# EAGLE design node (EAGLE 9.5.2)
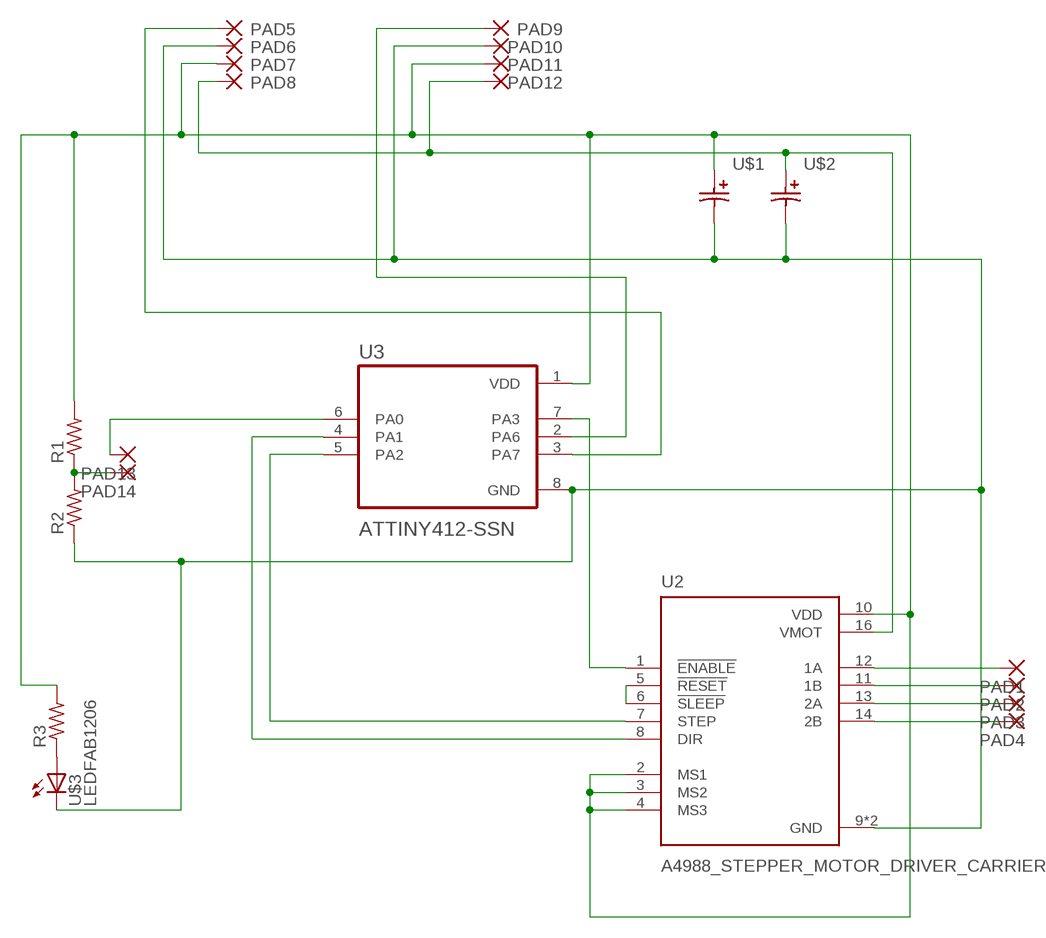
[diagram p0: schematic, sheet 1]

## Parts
PAD1  SMD2  [SMD1,27-2,54]
PAD2  SMD2  [SMD1,27-2,54]
PAD3  SMD2  [SMD1,27-2,54]
PAD4  SMD2  [SMD1,27-2,54]
PAD5  SMD2  [SMD1,27-2,54]
PAD6  SMD2  [SMD1,27-2,54]
PAD7  SMD2  [SMD1,27-2,54]
PAD8  SMD2  [SMD1,27-2,54]
PAD9  SMD2  [SMD1,27-2,54]
PAD10  SMD2  [SMD1,27-2,54]
PAD11  SMD2  [SMD1,27-2,54]
PAD12  SMD2  [SMD1,27-2,54]
PAD13  SMD2  [SMD1,27-2,54]
PAD14  SMD2  [SMD1,27-2,54]
R1  R1206FAB  [R1206FAB]
R2  R1206FAB  [R1206FAB]
R3  R1206FAB  [R1206FAB]
U2  A4988_STEPPER_MOTOR_DRIVER_CARRIER  [MODULE_A4988_STEPPER_MOTOR_DRIVER_CARRIER]
U3  ATTINY412-SSN  [SOIC127P600X175-8N]
U$1  CAP_POLARIZED  [SMD-ELEC-CAP]
U$2  CAP_POLARIZED  [SMD-ELEC-CAP]
U$3  LEDFAB1206  [LED1206FAB]

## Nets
N$1: PAD7.1(P) PAD11.1(P) R1.2 R3.2 U2.2(MS1) U2.3(MS2) U2.4(MS3) U2.10(VDD) U3.1(VDD) U$1.A
N$2: U2.5(!RESET) U2.6(!SLEEP)
N$3: R3.1 U$3.1(A)
N$4: U2.8(DIR) U3.4(PA1)
N$5: PAD13.1(P) U3.6(PA0)
N$6: PAD14.1(P) R1.1 R2.2
N$7: PAD6.1(P) PAD10.1(P) R2.1 U2.9(GND) U2.15(GND) U3.8(GND) U$1.C U$2.C U$3.2(C)
N$8: U2.1(!ENABLE) U3.7(PA3)
N$9: PAD5.1(P) U3.3(PA7)
N$13: U2.7(STEP) U3.5(PA2)
N$15: PAD8.1(P) PAD12.1(P) U2.16(VMOT) U$2.A
N$18: PAD1.1(P) U2.12(1A)
N$20: PAD2.1(P) U2.11(1B)
N$21: PAD3.1(P) U2.13(2A)
N$22: PAD4.1(P) U2.14(2B)
N$24: PAD9.1(P) U3.2(PA6)

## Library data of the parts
PAD1-PAD14 = wirepad:SMD2: SMD PAD
R1-R3 = fab:R: Resistor (US Symbol)
U2 = A4988_STEPPER_MOTOR_DRIVER_CARRIER_mod:A4988_STEPPER_MOTOR_DRIVER_CARRIER: Stepper motor controler; IC: A4988; 1A; Uin mot: 8÷35V; AVAILABILITY: Unavailable; DESCRIPTION: Stepper Motor Driver; MF: Pololu; MP: A4988 STEPPER MOTOR DRIVER CARRIER; PACKAGE: None; PRICE: None
U3 = ATTINY412-SSN:ATTINY412-SSN: None; AVAILABILITY: Unavailable; DESCRIPTION: AVR tinyAVR™ 1 Microcontroller IC 8-Bit 20MHz 4KB _4K x 8_ FLASH 8-SOIC; DIGIKEY-PURCHASE-URL: https://snapeda.com/shop?store=DigiKey&id=4002967; MF: Microchip Technology; MP: ATTINY412-SSN; PACKAGE: SOIC-8 Microchip Technology; PRICE: None
U$1 U$2 = fab:CAP_POLARIZED
U$3 = fab:LED: LED

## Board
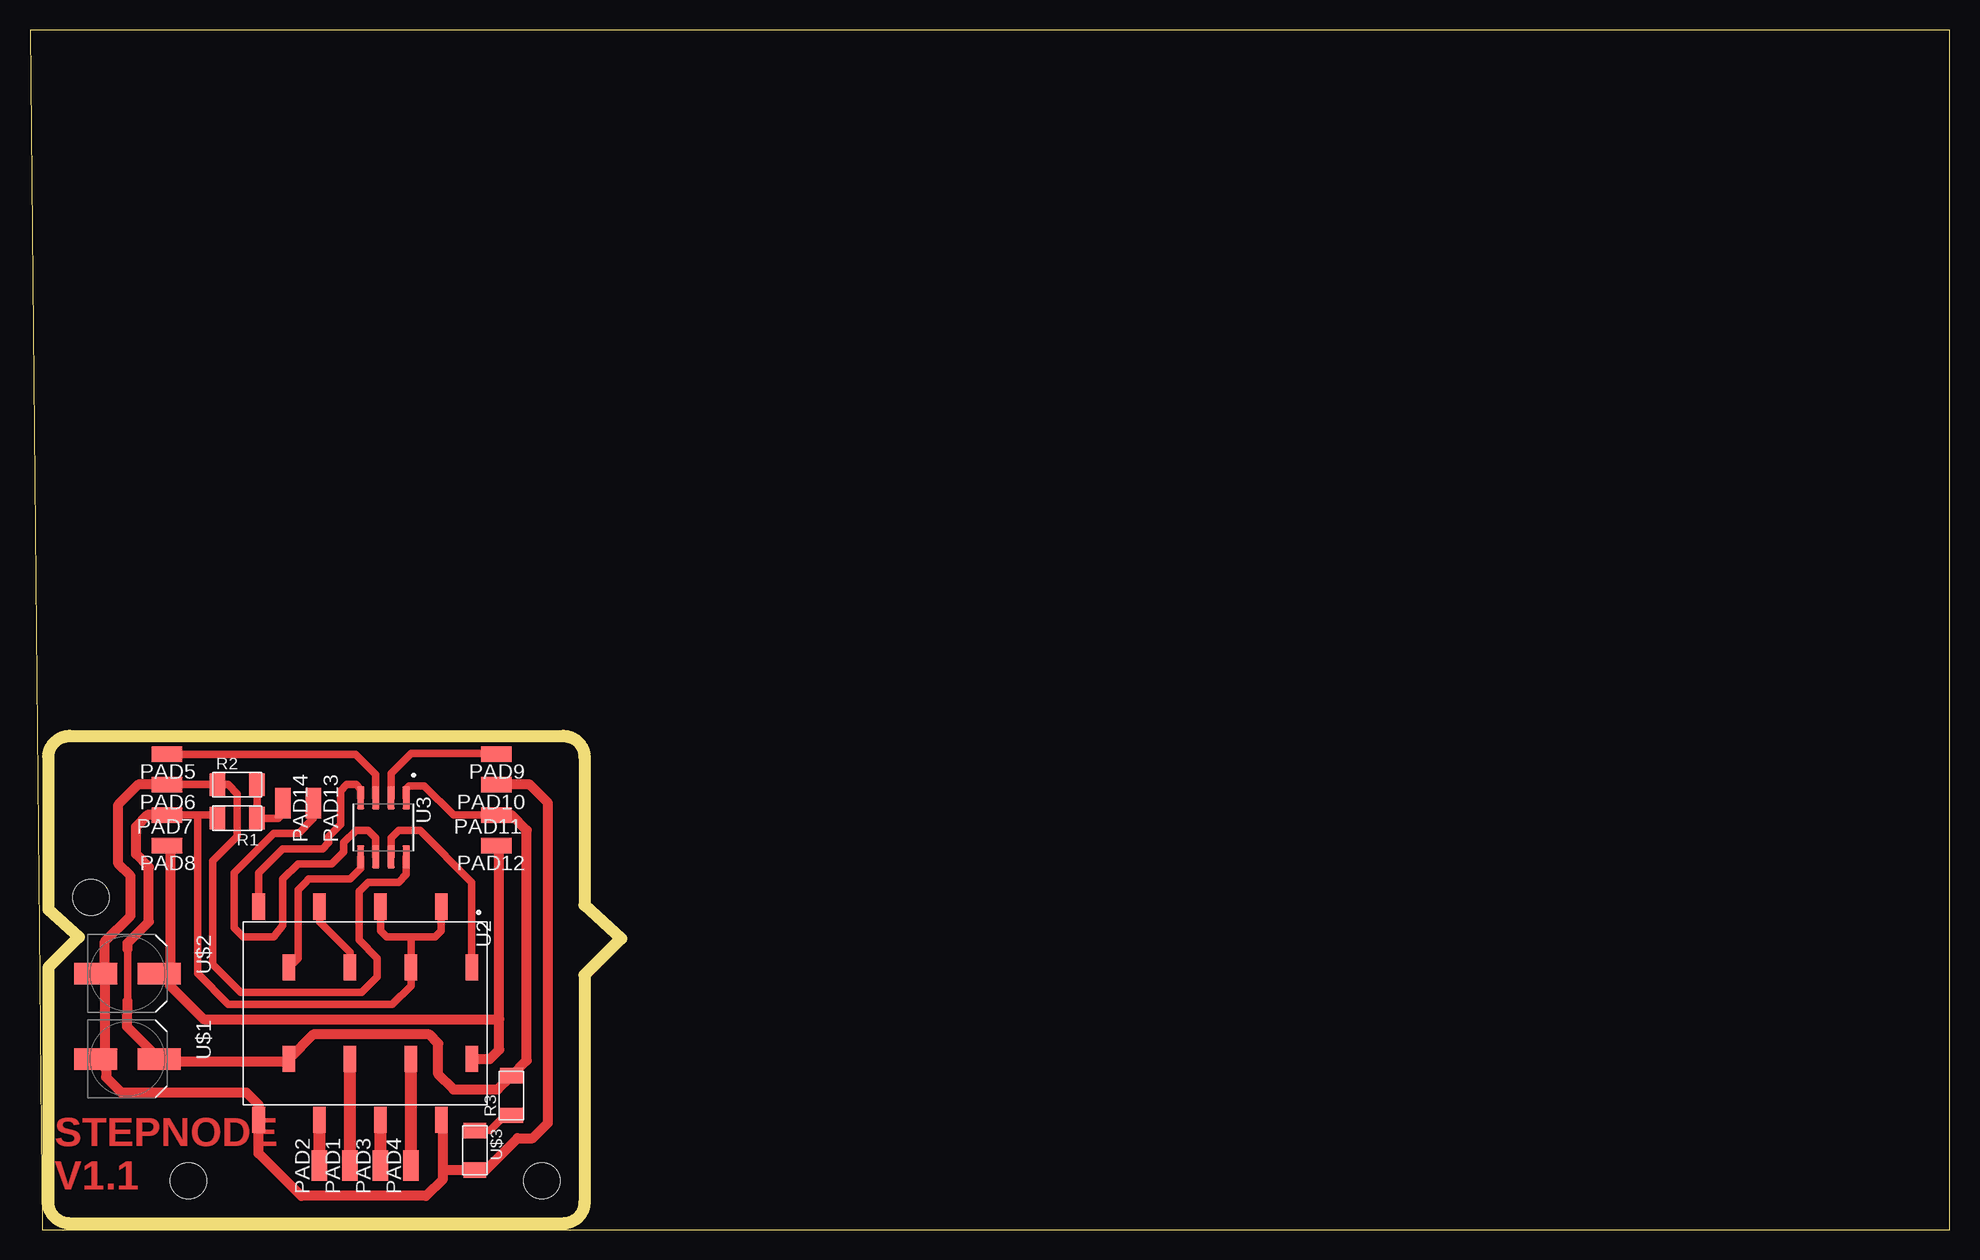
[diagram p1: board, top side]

Size 160 x 100 mm. Coordinates in mm from the lower left corner, seen from the top.
Outline: 1.02,0 160,0 160,100 0,100 1.02,0
Copper layers (1*16): Top 0.035mm / dielectric 1.5mm / Bottom 0.035mm
Design rules "default *": minimum track width 6mil, minimum drill 0.35mm, track to track 16mil, track to pad 16mil, pad to pad 16mil, via to via 16mil, smd to smd 16mil, copper to edge 40mil, drill to drill 6mil, minimum pad ring 10mil, minimum via ring 8mil, stop-mask expansion 4mil, vias tented up to drill 0mil, thermal gap 10mil
Holes 3 mm at 13.21,4.06 42.67,4.06 5.08,27.69
tKeepout: area 0.3,44.7 to 12.7,47
Milling: 14 lines

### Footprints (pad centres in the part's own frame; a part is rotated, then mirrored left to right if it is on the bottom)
SMD1,27-2,54 = smd 1.27 x 2.54: 1 0,0
R1206FAB = smd 1.27 x 1.905: 1 -1.651,0; 2 1.651,0
MODULE_A4988_STEPPER_MOTOR_DRIVER_CARRIER = smd 2.184 x 1.067: 1 -3.81,8.89; 2 -8.89,6.35; 3 -3.81,3.81; 4 -8.89,1.27; 5 -3.81,-1.27; 6 -8.89,-3.81; 7 -3.81,-6.35; 8 -8.89,-8.89; 9 8.89,-8.89; 10 3.81,-6.35; 11 8.89,-3.81; 12 3.81,-1.27; 13 8.89,1.27; 14 3.81,3.81; 15 8.89,6.35; 16 3.81,8.89
SOIC127P600X175-8N = smd 1.9 x 0.6: 1 -2.455,1.905; 2 -2.455,0.635; 3 -2.455,-0.635; 4 -2.455,-1.905; 5 2.455,-1.905; 6 2.455,-0.635; 7 2.455,0.635; 8 2.455,1.905
SMD-ELEC-CAP = smd 1.8 x 3.6: A 0,2.65; C 0,-2.65
LED1206FAB = smd 1.27 x 1.905: 1 -1.651,0; 2 1.651,0

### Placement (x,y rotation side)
PAD1  26.67,5.33 0 top
PAD2  24.13,5.33 0 top
PAD3  29.21,5.33 0 top
PAD4  31.75,5.33 0 top
PAD5  11.43,39.62 90 top
PAD6  11.43,37.08 90 top
PAD7  11.43,34.54 90 top
PAD8  11.43,32 90 top
PAD9  38.86,39.62 90 top
PAD10  38.86,37.08 90 top
PAD11  38.86,34.54 90 top
PAD12  38.86,32 90 top
PAD13  23.62,35.56 180 top
PAD14  21.08,35.56 180 top
R1  17.27,34.29 180 top
R2  17.27,37.08 0 top
R3  40.13,11.18 90 top
U2  27.94,18.03 270 top
U3  29.46,33.53 270 top
U$1  8.13,14.22 270 top
U$2  8.13,21.34 270 top
U$3  37.08,6.6 270 top

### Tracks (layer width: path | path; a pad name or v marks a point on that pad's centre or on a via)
N$1
  Top 0.61: U3.1 31.37,36.74 31.62,37 32.85,37 35.31,34.54 PAD11.1 | 31.75,24.38 29.72,24.38 29.21,24.89 U2.4 | 31.75,24.38 33.78,24.38 34.29,24.89 U2.2 | 31.75,24.38 U2.3 31.75,20.32 30.2,18.77 16.54,18.77 13.97,21.34 13.97,34.54 | 13.97,34.54 PAD7.1 | R1.2 15.37,34.54 13.97,34.54 | 8.13,19.05 8.13,23.37
  Top 0.813: PAD7.1 9.79,34.54 8.84,33.59 8.84,31.29 9.91,30.23 9.91,25.65 8.13,23.88 8.13,23.37 | 8.13,19.05 8.1,16.9 U$1.A 10.92,14.22 11.18,13.97 21.34,13.97 U2.10 23.62,16.26 33.27,16.26 34.04,15.49 34.04,12.95 35.31,11.68 38.99,11.68 R3.2 41.4,14.1 41.4,33.27 40.13,34.54 PAD11.1
N$2
  Top 0.61: U2.6 24.13,25.65 26.67,23.11 U2.5
N$3
  Top 0.61: R3.1 39.62,9.53 38.35,8.26 U$3.1
N$4
  Top 0.61: U2.8 19.05,29.72 21.08,31.75 24.38,31.75 24.89,32.26 24.89,32.77 25.91,33.78 25.91,36.58 26.42,37.08 27.18,37.08 27.56,36.7 U3.4
N$5
  Top 0.61: U3.6 28.83,32.64 28.19,33.27 27.18,33.27 26.16,32.26 26.16,31.5 25.15,30.48 22.35,30.48 21.08,29.21 21.08,25.34 20.32,24.38 17.78,24.38 17.02,25.15 17.02,29.72 20.32,33.02 22.39,33.02 23.62,34.25 PAD13.1
N$6
  Top 0.61: PAD14.1 21.08,34.67 20.7,34.29 R1.1 R2.2
N$7
  Top 0.61: PAD6.1 R2.1 16.51,37.08 17.27,36.32 17.27,32.77 15.24,30.73 15.24,22.1 17.55,19.79 27.66,19.79 28.96,21.08 28.96,22.61 27.43,24.13 27.43,28.19 28.19,28.96 30.73,28.96 31.37,29.59 U3.8
  Top 0.813: PAD6.1 9.03,37.08 7.37,35.42 7.37,30.48 8.38,29.46 8.38,26.16 6.24,24.02 6.24,22.1 U$2.C 6.24,20.57 6.24,14.99 U$1.C 6.35,13.35 6.35,12.7 7.62,11.43 18.03,11.43 19.05,10.41 U2.9 19.05,6.35 22.61,2.79 33.02,2.79 34.42,4.19 34.42,4.95 | PAD10.1 41.66,37.08 43.18,35.56 43.18,8.89 41.91,7.62 40.64,7.62 37.97,4.95 U$3.2 34.42,4.95 | 34.42,4.95 34.42,9.02 U2.15
N$8
  Top 0.61: U3.7 30.1,32.64 30.73,33.27 32.51,33.27 36.83,28.96 U2.1
N$9
  Top 0.61: U3.3 28.82,37.95 27.15,39.62 PAD5.1
N$13
  Top 0.61: U2.7 22.35,22.61 22.35,28.33 22.92,28.9 23.23,29.21 26.67,29.21 27.56,30.1 U3.5
N$15
  Top 0.61: PAD8.1 11.68,31.75 | U$2.A 11.68,21.34
  Top 0.813: U2.16 38.35,14.22 39.12,14.99 39.12,17.53 | PAD12.1 39.12,31.75 39.12,17.53 | 11.68,31.75 11.68,21.34 11.68,20.32 14.48,17.53 39.12,17.53
N$18
  Top 1.016: PAD1.1 U2.12
N$20
  Top 1.016: PAD2.1 U2.11
N$21
  Top 1.016: PAD3.1 U2.13
N$22
  Top 1.016: PAD4.1 U2.14
N$24
  Top 0.61: PAD9.1 38.79,39.7 31.78,39.7 30.1,38.02 U3.2

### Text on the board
Top: STEPNODE / V1.1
